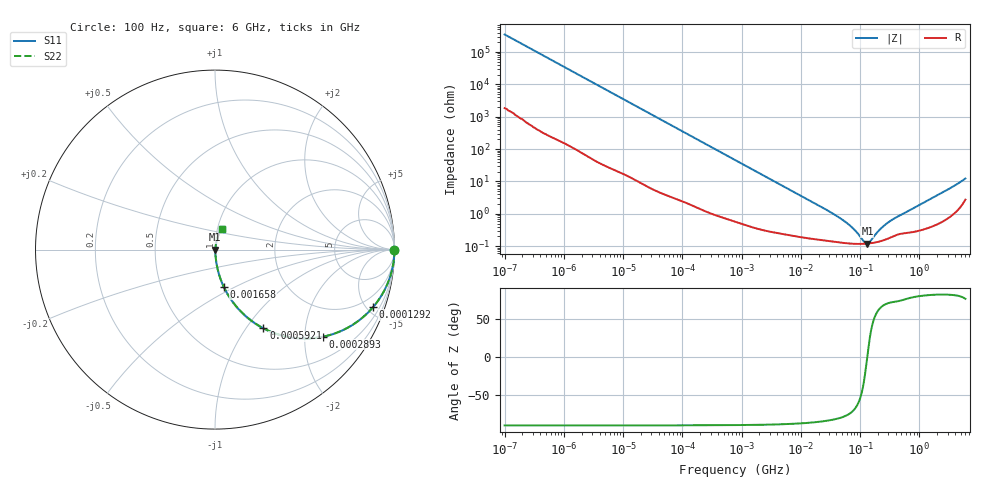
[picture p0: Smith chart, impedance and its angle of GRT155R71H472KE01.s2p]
!Murata Part Number: GRT155R71H472KE01
!These Parameters are Measured in Series Mode Connection
!Data Generated on Jun 19, 2026
!  o--ll--o
!Port1  Port2
!  o------o
!Operation Temp=25[degC], DC Bias Voltage=0[V]
!Freq. Start=100[Hz] Stop=6[GHz] 401[Steps]
# Hz S RI R 50
!Freq.(Hz) S11(Real) S11(Imag) S21(Real) S21(Imag) S12(Real) S12(Imag) S22(Real) S22(Imag)
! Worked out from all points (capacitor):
!   401 points, 100 Hz to 6 GHz, reference 50 ohm
!   read as one part in series: C = 4.56 nF near 109 Hz
!   lowest |Z| = 121 mohm at 133.4 MHz (marker M1)
!   series resonance near 132 MHz, so ESL is about 320 pH
!   S11 on the Smith chart (normalised r, x): 100 Hz: open; 129.2 kHz: 1.04, -5.50; 289.3 kHz: 1.02, -2.47; 592.1 kHz: 1.01, -1.21; 1.658 MHz: 1.01, -0.43; 6 GHz: 1.05, +0.24
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100  1 -0.000287  1.6e-06 0.000287  1.6e-06 0.000287  1 -0.000287
2008  0.9999 -0.00572  5.74e-05 0.00572  5.74e-05 0.00572  0.9999 -0.00572
12592  0.9986 -0.0356  0.00145 0.0356  0.00145 0.0356  0.9986 -0.0356
40335  0.9866 -0.1123  0.0134 0.1123  0.0134 0.1123  0.9866 -0.1123
129199  0.8816 -0.3195  0.1184 0.3195  0.1184 0.3195  0.8816 -0.3195
193316  0.7707 -0.4165  0.2293 0.4165  0.2293 0.4165  0.7707 -0.4165
289253  0.6026 -0.4851  0.3974 0.4851  0.3974 0.4851  0.6026 -0.4851
413847  0.4278 -0.49  0.5722 0.49  0.5722 0.49  0.4278 -0.49
592111  0.27 -0.4384  0.73 0.4384  0.73 0.4384  0.27 -0.4384
774597  0.1795 -0.3776  0.8205 0.3776  0.8205 0.3776  0.1795 -0.3776
1658239  0.0482 -0.206  0.9518 0.206  0.9518 0.206  0.0482 -0.206
4246196  0.00967 -0.0843  0.9903 0.0843  0.9903 0.0843  0.00967 -0.0843
1.555665e7  0.00222 -0.0233  0.9978 0.0233  0.9978 0.0233  0.00222 -0.0233
5.699437e7  0.00127 -0.00542  0.9987 0.00542  0.9987 0.00542  0.00127 -0.00542
8.154455e7  0.00119 -0.0029  0.9988 0.0029  0.9988 0.0029  0.00119 -0.0029
1.166697e8  0.00118 -0.000716  0.9988 0.000716  0.9988 0.000716  0.00118 -0.000716
1.334425e8  0.0012 6.61e-05  0.9988 -6.61e-05  0.9988 -6.61e-05  0.0012 6.61e-05
1.459435e8  0.00122 0.000586  0.9988 -0.000586  0.9988 -0.000586  0.00122 0.000586
2.283698e8  0.00145 0.00331  0.9985 -0.00331  0.9985 -0.00331  0.00145 0.00331
3.124326e8  0.00181 0.00545  0.9982 -0.00545  0.9982 -0.00545  0.00181 0.00545
1.95892e9  0.00587 0.0356  0.9941 -0.0356  0.9941 -0.0356  0.00587 0.0356
6e9  0.0399 0.1126  0.9601 -0.1126  0.9601 -0.1126  0.0399 0.1126
